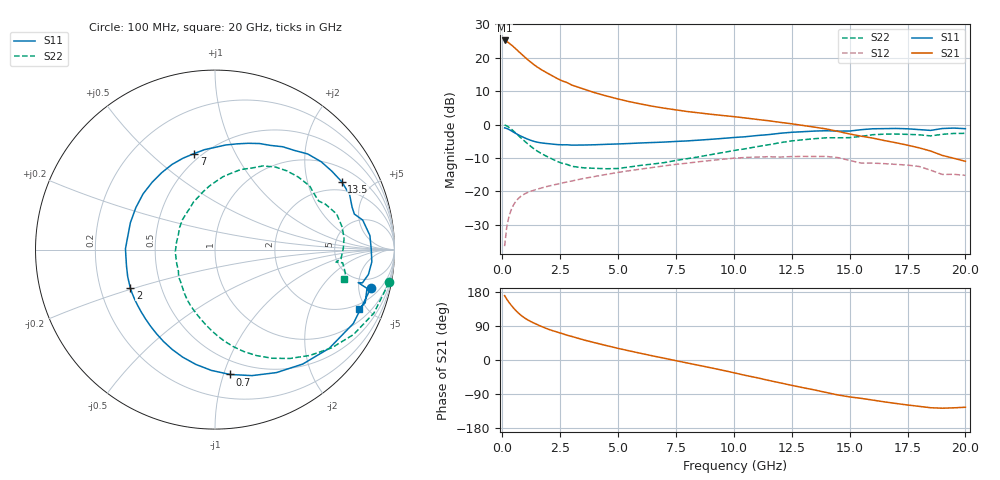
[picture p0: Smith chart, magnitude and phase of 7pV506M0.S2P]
! Infineon Technologies  Discrete & RF Semiconductors
! bfp620
! VCE = 0.50 V,  IC =  6.0 mA
! Common Emitter S-Parameters:  Sep 2002
# GHz  S  MA  R  50
!  f  S11  S21  S12  S22
! GHz  MAG  ANG  MAG  ANG  MAG  ANG  MAG  ANG
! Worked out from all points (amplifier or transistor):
!   59 points, 100 MHz to 20 GHz, reference 50 ohm
!   highest |S21| = 25.2 dB at 100 MHz (marker M1)
!   |S21| within 3 dB of that: start of sweep to 658.3 MHz
!   unconditionally stable (mu >= 1): 4.531 GHz to 10.43 GHz; 17.06 GHz to end of sweep
!   at 1 GHz: K = 0.38, MSG = 20.3 dB, |S12| = -20.6 dB
!   at 5.5 GHz: K = 1.05, MAG = 9.0 dB, |S12| = -13.8 dB
!   at 20 GHz: K = 1.74, MAG = -2.9 dB, |S12| = -15.2 dB
!   S11 on the Smith chart (normalised r, x): 100 MHz: 3.21, -6.85; 700 MHz: 0.38, -1.05; 2 GHz: 0.33, -0.19; 7 GHz: 0.46, +0.70; 13.5 GHz: 1.56, +3.29; 20 GHz: 1.66, -4.48
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0.1  0.8952 -13.7  18.23 169.8  0.0151 79.8  0.9871 -10.7
0.2  0.8739 -28.1  17.51 159.8  0.0307 74.5  0.9534 -21.8
0.3  0.8413 -40.8  16.57 151.1  0.0436 68.3  0.9054 -31.5
0.4  0.8036 -52.5  15.54 143.3  0.0547 62.5  0.8498 -40.1
0.5  0.7662 -63.4  14.49 136.1  0.064 57.5  0.7921 -48.1
0.6  0.7318 -73.6  13.47 129.6  0.072 53.2  0.7361 -55.5
0.7  0.7009 -83.1  12.52 123.7  0.0787 49.5  0.6836 -62.3
0.8  0.6734 -91.7  11.63 118.4  0.0843 46.3  0.6352 -68.5
0.9  0.6484 -99.5  10.81 113.7  0.089 43.6  0.5911 -74.1
1  0.6257 -106.7  10.07 109.5  0.093 41.4  0.5509 -79.2
1.2  0.5866 -119.3  8.787 102.5  0.0995 37.8  0.4818 -88.2
1.4  0.5574 -130.2  7.761 96.5  0.105 35.3  0.4266 -96.2
1.6  0.5383 -139.7  6.957 90.9  0.1101 33.3  0.384 -103.7
2  0.5178 -155.8  5.776 81.0  0.1199 30.4  0.324 -117.8
2.6  0.4979 -175.3  4.503 69.4  0.1337 26.9  0.2625 -136.9
3.5  0.4947 162.4  3.426 53.3  0.1557 21.8  0.2256 -162.6
5  0.5131 133.1  2.42 30.7  0.1923 12.4  0.2202 158.2
7  0.5477 102.2  1.762 4.6  0.2412 -2.5  0.2699 121.2
10.5  0.6584 61.8  1.257 -40.6  0.3222 -36.8  0.4349 78.0
13.5  0.8009 28.2  0.915 -79.2  0.3329 -69.5  0.6157 41.0
17  0.8764 -4.5  0.535 -114.7  0.2536 -100.4  0.7216 4.9
20  0.8689 -22.3  0.282 -124.7  0.1738 -114.1  0.7402 -13.0
